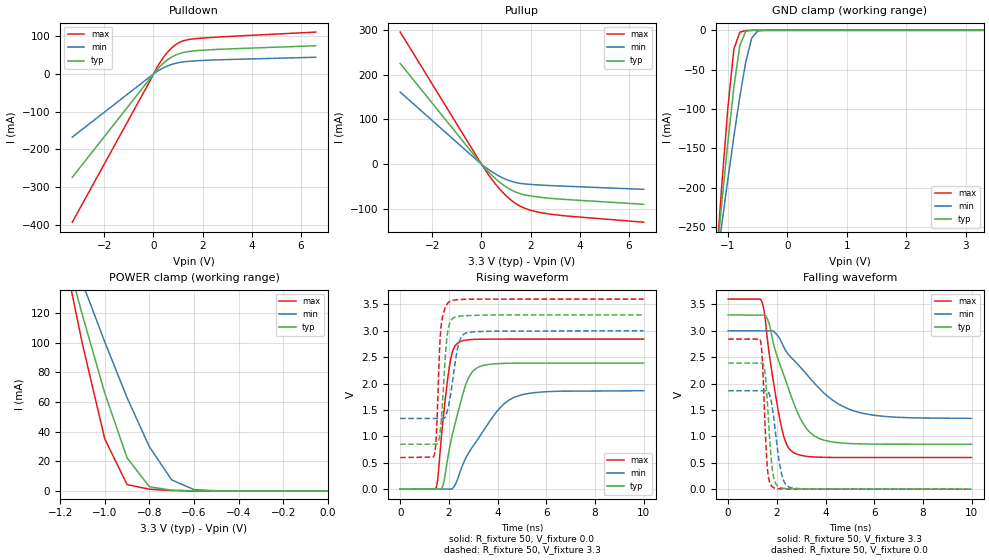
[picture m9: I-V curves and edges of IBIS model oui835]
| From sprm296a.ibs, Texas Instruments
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[Model]   oui835
Model_type   3-state
Enable   Active-Low
Polarity   Non-Inverting
| signals   A, GZ, Y
Vmeas = 1.5
|   typ   min   max
C_comp   3.857p   3.787p   3.900p
|   typ   min   max
[Temperature Range]   25   -40   125
|   typ   min   max
[Voltage Range]   3.30V   3.00V   3.60V
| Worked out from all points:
|   slope of the pulldown table from 0 to 0.495 V, typ, clamps not added: 14.6 ohm
|   slope of the pullup table from 0 to 0.495 V, typ, clamps not added: 17.1 ohm
|   GND clamp passes 1 mA (typ) near -0.69 V on its own axis
|   POWER clamp passes 1 mA (typ) near -0.72 V on its own axis
|   rising waveform, R_fixture 50, V_fixture 0.0: 20-80 % time 729ps typ, 1.52ns min, 391ps max; typ from 0 V to 2.39 V
|   falling waveform, R_fixture 50, V_fixture 3.3: 20-80 % time 1.13ns typ, 2.02ns min, 605ps max; typ from 3.3 V to 0.851 V
|   rising waveform, R_fixture 50, V_fixture 3.3: 20-80 % time 213ps typ, 335ps min, 160ps max; typ from 0.851 V to 3.3 V
|   falling waveform, R_fixture 50, V_fixture 0.0: 20-80 % time 217ps typ, 326ps min, 161ps max; typ from 2.39 V to 0 V
[Pulldown]
|   Voltage   I(typ)   I(min)   I(max)
-3.3V     -273.9mA   -167.3mA   -393.2mA
-200mV    -17mA      -10.01mA   -25.19mA
200mV     15.78mA    9.018mA    24.02mA
500mV     34.27mA    19.55mA    52.44mA
700mV     43.5mA     24.72mA    66.87mA
900mV     50.47mA    28.56mA    77.95mA
1.2V      57.14mA    32.16mA    88.1mA
1.8V      62.45mA    35.48mA    94.53mA
6.6V      75.19mA    44.76mA    111.5mA
[GND_clamp]
|   Voltage   I(typ)   I(min)   I(max)
-3.3V     -2.083A    -1.584A    -2.679A
-1.2V     -296.2mA   -302.6mA   -298.4mA
-1.1V     -217.5mA   -245.3mA   -194.6mA
-1V       -142mA     -189.4mA   -98.34mA
-900mV    -72.82mA   -135.4mA   -24.18mA
-800mV    -19.4mA    -84.68mA   -2.46mA
-700mV    -1.167mA   -40.37mA   -232.9uA
-600mV    -46.46uA   -10.03mA   -13.1uA
-500mV    -2.237uA   -877.9uA   -453nA
-300mV    -4.185nA   -2.882uA   -532.9pA
3.3V      222pA      870.1nA    266.4pA
[Pullup]
|   Voltage   I(typ)   I(min)   I(max)
-3.3V     224.7mA    160.6mA    295mA
100mV     -6.373mA   -4.422mA   -8.632mA
400mV     -23.87mA   -16.43mA   -32.51mA
700mV     -38.83mA   -26.47mA   -53.25mA
1.2V      -57.64mA   -38.47mA   -80.36mA
1.5V      -65mA      -42.63mA   -91.89mA
1.8V      -69.49mA   -44.77mA   -99.81mA
2.5V      -75.13mA   -47.46mA   -109.6mA
3.5V      -79.61mA   -49.93mA   -116.5mA
6.6V      -90.17mA   -56.73mA   -130.2mA
[POWER_clamp]
|   Voltage   I(typ)   I(min)   I(max)
-3.3V     1.452A     1.103A     1.872A
-1.2V     174.2mA    181.2mA    171.9mA
-1.1V     118.4mA    140.2mA    98.96mA
-1V       65.96mA    100.4mA    35.03mA
-900mV    22.27mA    62.84mA    4.252mA
-800mV    2.8mA      29.73mA    1.177mA
-700mV    510.2uA    7.413mA    243.5uA
-600mV    79.93uA    885.8uA    20.02uA
-500mV    6.747uA    98.94uA    768.8nA
0V        1pA        1pA        1pA
[Ramp]
|   I(typ)   I(min)   I(max)
dV/dt_r   1.433/0.728n   1.118/1.512n   1.706/0.390n
dV/dt_f   1.469/1.130n   0.996/2.023n   1.801/0.603n
[Rising Waveform]
R_fixture = 50
V_fixture = 0.0
|  pu_on
|  TIME   V(typ)   V(min)   V(max)
0s        2nV        6nV        2nV
1.485ns   816.3uV    1.216mV    35.74mV
1.756ns   65.59mV    1.216mV    1.302V
2.027ns   789mV      1.216mV    2.347V
2.19ns    1.123V     33.42mV    2.655V
2.407ns   1.516V     259.3mV    2.78V
3.004ns   2.242V     823.2mV    2.836V
4.089ns   2.379V     1.535V     2.842V
4.686ns   2.386V     1.74V      2.842V
10ns      2.388V     1.864V     2.842V
[Falling Waveform]
R_fixture = 50
V_fixture = 3.3
V_fixture_min = 3.0
V_fixture_max = 3.6
|  pd_on
|  TIME   V(typ)   V(min)   V(max)
0s        3.3V       3V         3.6V
1.394ns   3.296V     2.997V     3.543V
1.529ns   3.296V     2.997V     3.199V
1.665ns   3.158V     2.997V     2.64V
2.139ns   2.35V      2.834V     1.286V
2.41ns    1.994V     2.593V     839.6mV
2.68ns    1.645V     2.45V      695.5mV
3.493ns   1.024V     2.032V     611.3mV
5.185ns   861.3mV    1.479V     599.3mV
10ns      851.4mV    1.34V      599.1mV
[Rising Waveform]
R_fixture = 50
V_fixture = 3.3
V_fixture_min = 3.0
V_fixture_max = 3.6
|  pd_off
|  TIME   V(typ)   V(min)   V(max)
0s        851.4mV    1.339V     599.1mV
1.41ns    851.4mV    1.339V     666.1mV
1.488ns   851.4mV    1.339V     1.069V
1.618ns   1.018V     1.339V     2.678V
1.67ns    1.226V     1.339V     3.055V
1.879ns   2.679V     1.401V     3.469V
2.035ns   3.147V     1.699V     3.557V
2.373ns   3.272V     2.697V     3.589V
2.685ns   3.285V     2.954V     3.595V
10ns      3.3V       3V         3.6V
[Falling Waveform]
R_fixture = 50
V_fixture = 0.0
|  pu_off
|  TIME   V(typ)   V(min)   V(max)
0s        2.388V     1.864V     2.842V
1.316ns   2.388V     1.863V     2.835V
1.412ns   2.388V     1.863V     2.381V
1.508ns   2.232V     1.863V     1.309V
1.604ns   1.698V     1.862V     442mV
1.757ns   632.7mV    1.692V     77.78mV
1.853ns   261.5mV    1.415V     33.15mV
2.197ns   24.75mV    281.7mV    6.724mV
2.523ns   8.206mV    36.34mV    3.164mV
10ns      74.49nV    5.112uV    44.9nV
